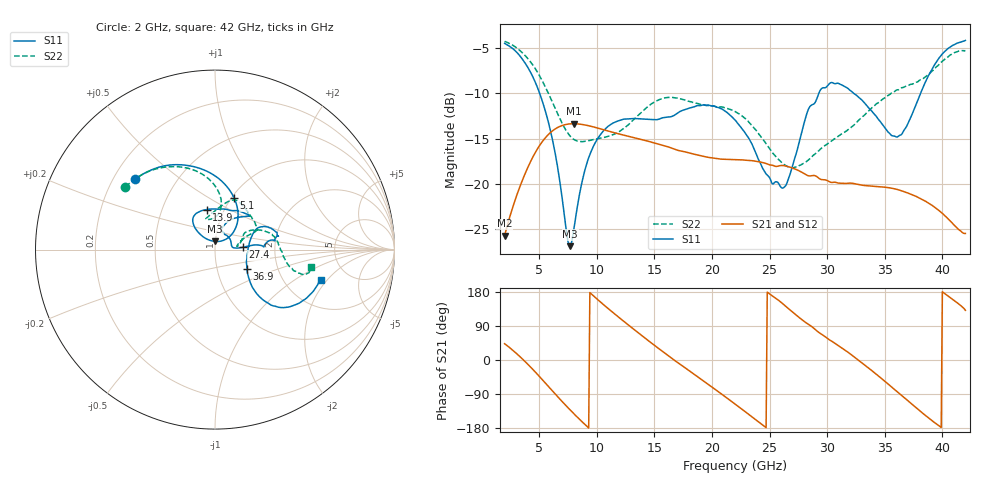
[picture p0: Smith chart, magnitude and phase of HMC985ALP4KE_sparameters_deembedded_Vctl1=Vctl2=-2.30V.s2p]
!s2p File: Measurements: S11, S21, S12, S22
# GHz S dB R 50.0
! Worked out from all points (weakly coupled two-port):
!   401 points, 2 GHz to 42 GHz, reference 50 ohm
!   highest |S21| = -13.36 dB at 8 GHz (marker M1); lowest = -25.7 dB at 2 GHz (marker M2)
!   lowest |S11| = -26.8 dB at 7.7 GHz (marker M3), VSWR 1.10, Z = 49.8 + j4.55 ohm
!   |S11| at or under -10 dB: 5.034 GHz to 29.29 GHz (24.25 GHz wide, 141 % of centre); 32.28 GHz to 38.12 GHz (5.837 GHz wide, 16.6 % of centre)
!   |S22| runs from -18.2 to -4.3 dB; largest |S21 - S12| = 0.0002
!   S11 on the Smith chart (normalised r, x): 2 GHz: 0.29, +0.35; 5.1 GHz: 1.03, +0.65; 13.9 GHz: 0.83, +0.39; 27.4 GHz: 1.36, +0.03; 36.9 GHz: 1.39, -0.31; 42 GHz: 3.19, -1.73
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2  -4.53 138.7  -25.67 43.0  -25.68 43.0  -4.31 145.0
3.5  -6.20 107.4  -19.73 4.1  -19.73 4.1  -5.52 119.5
5.1  -10.24 69.9  -15.65 -46.1  -15.65 -46.1  -8.25 93.9
6.2  -15.40 46.8  -14.11 -83.2  -14.11 -83.2  -11.13 82.9
7.7  -26.83 89.8  -13.38 -132.2  -13.38 -132.2  -14.74 88.5
8  -25.08 115.3  -13.36 -141.4  -13.37 -141.4  -15.09 92.1
8.7  -19.88 133.3  -13.44 -162.3  -13.45 -162.3  -15.34 99.9
10.7  -13.99 128.2  -14.06 143.2  -14.07 143.1  -14.86 105.9
13.9  -12.84 101.6  -15.11 64.7  -15.12 64.7  -12.08 81.2
15.4  -12.87 82.9  -15.63 29.7  -15.63 29.7  -10.73 71.3
19  -11.38 45.4  -16.88 -49.4  -16.89 -49.4  -11.25 45.1
22  -12.95 53.4  -17.32 -116.2  -17.33 -116.2  -12.03 24.4
24.5  -18.48 72.4  -17.67 -173.9  -17.67 -173.9  -15.21 21.3
26.1  -20.46 15.1  -17.96 149.6  -17.96 149.6  -17.69 12.8
27.4  -16.26 4.7  -18.45 116.3  -18.45 116.3  -18.12 8.3
28.7  -11.28 3.2  -19.07 87.2  -19.09 87.2  -16.96 13.3
31.1  -9.01 16.0  -19.90 35.3  -19.92 35.3  -14.63 28.8
33.3  -11.17 26.7  -20.17 -14.1  -20.17 -14.1  -12.35 26.7
35.4  -14.41 7.2  -20.41 -66.3  -20.42 -66.3  -10.18 18.1
36.9  -13.65 -31.4  -20.94 -104.8  -20.94 -104.9  -9.20 9.2
39.7  -6.17 -41.1  -22.91 -173.5  -22.91 -173.6  -6.87 -15.0
42  -4.21 -15.9  -25.44 131.0  -25.45 131.0  -5.32 -10.1
